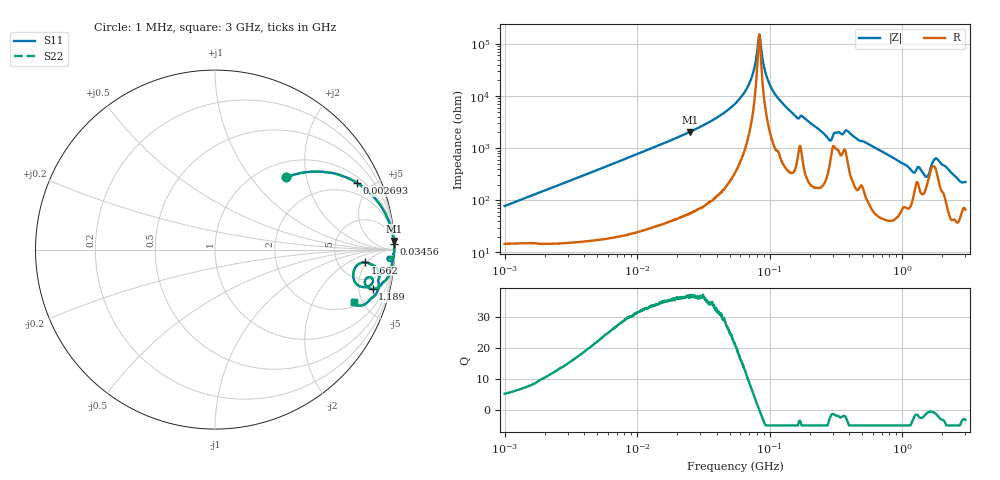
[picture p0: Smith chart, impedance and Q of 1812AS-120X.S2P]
!s-Parameter Generated by FASTRON Sdn. Bhd.
!FASTRON P/N : 1812AS-120X
!Keysight Technologies,E4991B,MY54100416,A.01.15
!Date created: Mon Oct 16 09:37:50 2023
!Version  : Rev00 Mon Oct 16 09:37:50 2023
!Data & Calibration Information:
!Freq	S11	S21	S12	S22
!PortZ  Port1:50+j0  Port2:50+j0
!When reading, reference impedance value at option line is always used.
! Remarks : This data is being provided solely for informational purposes.
# Hz S dB R 50
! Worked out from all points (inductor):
!   1601 points, 1 MHz to 3 GHz, reference 50 ohm
!   read as one part in series: L = 12.1 uH near 1.041 MHz
!   highest Q = 36.7 at 24.97 MHz (marker M1), where L = 13 uH
!   self-resonance near 83.39 MHz
!   S11 on the Smith chart (normalised r, x): 1 MHz: 1.29, +1.53; 2.693 MHz: 1.30, +4.10; 34.56 MHz: 3, +62; 1.189 GHz: 2.86, -6.98; 1.662 GHz: 9, -5; 3 GHz: 2.33, -4.28
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1000000  -4.97 45.5  -2.78 -33.7  -2.78 -33.7  -4.97 45.5
2693356  -1.16 25.1  -7.42 -60.7  -7.42 -60.7  -1.16 25.1
3804036  -0.63 18.7  -9.88 -68.2  -9.88 -68.2  -0.63 18.7
1.447069e7  -0.06 5.1  -21.06 -83.2  -21.06 -83.2  -0.06 5.1
2.49671e7  -0.02 2.8  -26.24 -85.7  -26.24 -85.7  -0.02 2.8
3.456417e7  -0.01 1.8  -29.84 -86.5  -29.84 -86.5  -0.01 1.8
5.477226e7  -0.01 0.8  -37.01 -86.4  -37.01 -86.4  -0.01 0.8
7.105049e7  -0.01 0.3  -45.45 -82.8  -45.45 -82.8  -0.01 0.3
8.380746e7  -0.01 -0.0  -63.61 7.6  -63.61 7.6  -0.01 -0.0
9.450168e7  -0.01 -0.2  -47.75 79.7  -47.75 79.7  -0.01 -0.2
1.092603e8  -0.01 -0.5  -40.84 84.1  -40.84 84.1  -0.01 -0.5
1.582265e8  -0.03 -1.4  -32.07 82.2  -32.07 82.2  -0.03 -1.4
2.083556e8  -0.02 -2.0  -29.21 84.3  -29.21 84.3  -0.02 -2.0
2.813178e8  -0.19 -3.7  -23.39 69.2  -23.39 69.2  -0.19 -3.7
3.836505e8  -0.12 -2.5  -26.84 70.6  -26.84 70.6  -0.12 -2.5
7.925923e8  -0.14 -7.7  -17.43 79.1  -17.43 79.1  -0.14 -7.7
1.188719e9  -0.86 -14.0  -12.01 61.1  -12.01 61.1  -0.86 -14.0
1.333714e9  -0.98 -10.7  -13.74 53.7  -13.74 53.7  -0.98 -10.7
1.519029e9  -1.96 -12.8  -10.92 38.5  -10.92 38.5  -1.96 -12.8
1.662201e9  -1.52 -4.9  -14.97 23.8  -14.97 23.8  -1.52 -4.9
1.818868e9  -0.79 -6.9  -16.79 49.7  -16.79 49.7  -0.79 -6.9
3e9  -1.65 -20.6  -8.66 52.2  -8.66 52.2  -1.65 -20.6
